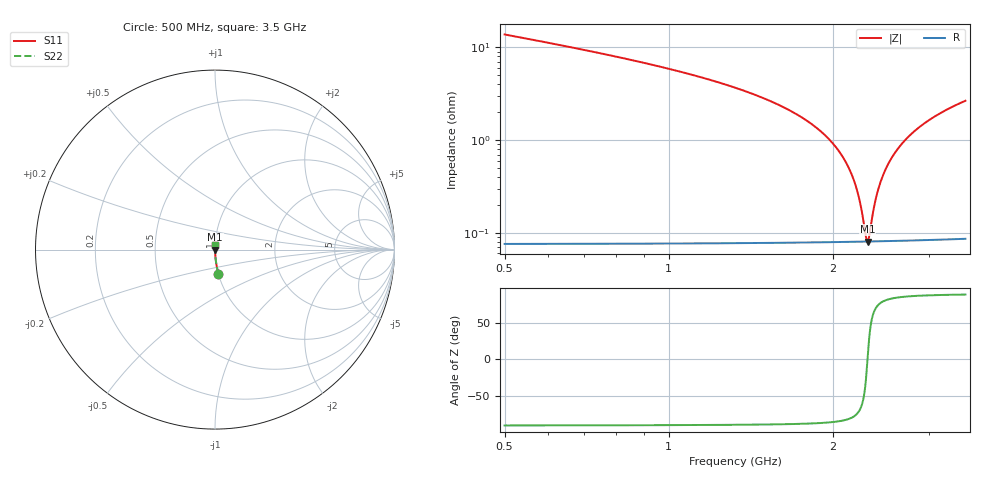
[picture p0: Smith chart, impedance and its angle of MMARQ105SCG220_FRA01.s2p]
! MMARQ105SCG220_FRA01  S-PARAMETER MODEL  ( General Type )
! Model Generated by TAIYO YUDEN Corporation (http://www.ty-top.com)
! Version 1.0
! TAIYO YUDEN Control No. 200326
! Copyright(c) 2020 TAIYO YUDEN CO.,LTD. All Rights Reserved.
! Product Description (link to TY-COMPAS)
! https://ds.yuden.co.jp/TYCOMPAS/or/detail?pn=MMARQ105SCG220JFRA01&u=M
! Products Name : Multilayer Ceramic Capacitors
! Characteristics :
!  Capacitance : 22 pF , Rated Voltage : 250V , TCC : CG / C0G
!  Case Size : 1.0 x 0.5 / 0.039 x 0.02 [mm/inch] , Thickness : 0.5 / 0.02 [mm/inch]
!  (Conditions: Temperature = 25 degC , DC Bias Current/Voltage = 0A / 0V)
! External Node Assignments :
!  1  o---| |---o  2
! GND o---------o GND
! Frequency Range : 500MHz  -  3.5GHz  [ 401 STEP ]
# MHz S RI R 50
! Freq[MHz].  S11 Real  S11 Imag  S21 Real  S21 Imag  S12 Real  S12 Imag  S22 Real  S22 Imag
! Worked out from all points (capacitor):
!   401 points, 500 MHz to 3.5 GHz, reference 50 ohm
!   read as one part in series: C = 22 pF near 515 MHz
!   lowest |Z| = 80.6 mohm at 2.315 GHz (marker M1)
!   series resonance near 2.315 GHz, so ESL is about 220 pH
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500  0.0194 -0.1353  0.9806 0.1353  0.9806 0.1353  0.0194 -0.1353
725  0.00879 -0.0892  0.9912 0.0892  0.9912 0.0892  0.00879 -0.0892
1002.5  0.00419 -0.0584  0.9958 0.0584  0.9958 0.0584  0.00419 -0.0584
1505  0.00155 -0.0277  0.9985 0.0277  0.9985 0.0277  0.00155 -0.0277
1797.5  0.00104 -0.016  0.999 0.016  0.999 0.016  0.00104 -0.016
2000  0.000878 -0.00916  0.9991 0.00916  0.9991 0.00916  0.000878 -0.00916
2105  0.000833 -0.00595  0.9992 0.00595  0.9992 0.00595  0.000833 -0.00595
2187.5  0.000813 -0.00354  0.9992 0.00354  0.9992 0.00354  0.000813 -0.00354
2232.5  0.000807 -0.00227  0.9992 0.00227  0.9992 0.00227  0.000807 -0.00227
2255  0.000806 -0.00164  0.9992 0.00164  0.9992 0.00164  0.000806 -0.00164
2300  0.000805 -0.000405  0.9992 0.000405  0.9992 0.000405  0.000805 -0.000405
2315  0.000805 6.47e-07  0.9992 -6.47e-07  0.9992 -6.47e-07  0.000805 6.47e-07
2330  0.000806 0.000404  0.9992 -0.000404  0.9992 -0.000404  0.000806 0.000404
2375  0.00081 0.0016  0.9992 -0.0016  0.9992 -0.0016  0.00081 0.0016
2412.5  0.000816 0.00258  0.9992 -0.00258  0.9992 -0.00258  0.000816 0.00258
2450  0.000824 0.00354  0.9992 -0.00354  0.9992 -0.00354  0.000824 0.00354
2502.5  0.000837 0.00487  0.9992 -0.00487  0.9992 -0.00487  0.000837 0.00487
2592.5  0.000867 0.00708  0.9991 -0.00708  0.9991 -0.00708  0.000867 0.00708
2697.5  0.000914 0.00958  0.9991 -0.00958  0.9991 -0.00958  0.000914 0.00958
2832.5  0.000989 0.0127  0.999 -0.0127  0.999 -0.0127  0.000989 0.0127
3005  0.00111 0.0165  0.9989 -0.0165  0.9989 -0.0165  0.00111 0.0165
3500  0.00157 0.0265  0.9984 -0.0265  0.9984 -0.0265  0.00157 0.0265
